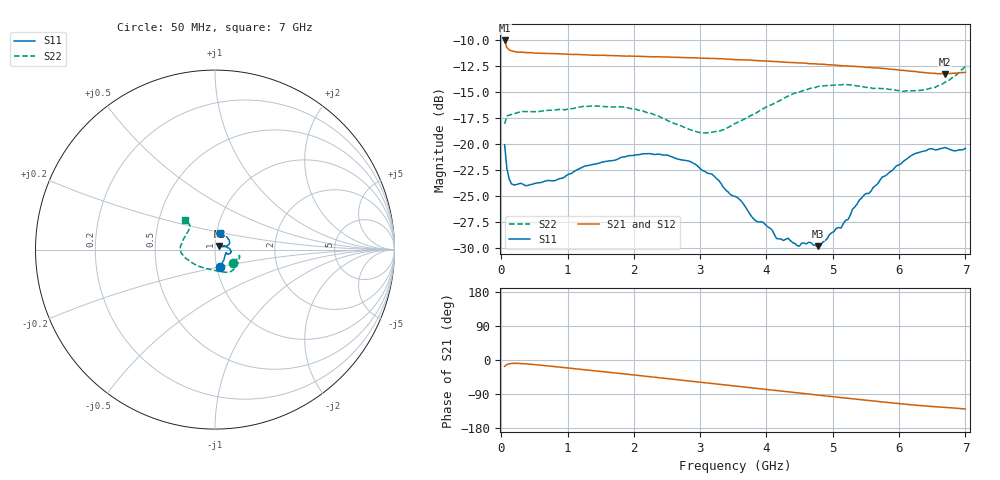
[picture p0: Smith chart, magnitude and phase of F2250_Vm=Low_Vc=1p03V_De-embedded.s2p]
! Integrated Device Technology
! Corporate Headquarters
! 6024 Silver Creek Valley Road
! San Jose, CA 95138  USA
! Phone:  1-408-284-8200
! Toll Free:  1-800-223-1366
! Webpage:  http://www.idt.com/
! Timing and RF Division
! 515 Groton Road, Suite 102
! Westford, MA 01886-6024
! Device:  F2250
! Description: Voltage Variable RF Attenuator
! Frequency:  50.0 -  6000.00 MHz
! Package:  3x3 mm Thin QFN Plastic Package: 16 pin
! Ports:  2 RF, 3 DC
!  Pin  1  = GND
!  Pin  2  = NC
!  Pin  3  = RF1  = Port 1
!  Pin  4  = NC
!  Pin  5  = GND
!  Pin  6  = GND
!  Pin  7  = GND
!  Pin  8  = GND
!  Pin  9  = NC
!  Pin 10  = RF2  = Port 2
!  Pin 11  = NC
!  Pin 12  = GND
!  Pin 13  = GND
!  Pin 14  = VCNTRL
!  Pin 15  = VDD
!  Pin 16  = VMODE
! Vcntrl:  1.030 Volts
! Vmode:  +0.000 Volts
! Vdd:  +3.30  Volts
! Current:  1.188 mA
! Data:  The device was measured on a the F2250 evaluation board which has
!  individual transmission lines to the RF pins.  Data was collected
!  using a calibrated network analyzer.  The evaluation board was
!  de-embedded using a TRL calibration technique.
!  The reference plane is the edge of the package pin.
! Misc:  SN 10
!  Action Tracker AT0258
! Date Measured:  2014-11-26
! Date:  2015-10-15  MJV
! Note:
!  Integrated Device Technology supplies this data as a sample of measured
!  data at the package pin for this product.  Your particular data for this
!  product may vary.
!  Data was taken at 25 degrees C.
!  Integrated Device Technology reserves the right to change this data at anytime.
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# GHz S dB R 50
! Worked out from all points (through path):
!   201 points, 50 MHz to 7 GHz, reference 50 ohm
!   highest |S21| = -10.00 dB at 50 MHz (marker M1); lowest = -13.2 dB at 6.687 GHz (marker M2)
!   group delay of S21, straight-line fit = 51.3 ps
!   lowest |S11| = -29.8 dB at 4.776 GHz (marker M3), VSWR 1.07, Z = 52.5 + j2.14 ohm
!   |S11| at or under -10 dB: start of sweep to end of sweep
!   |S22| runs from -18.9 to -12.5 dB; largest |S21 - S12| = 0.00076
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0.05  -20.05 -73.6  -10.00 -16.6  -10.01 -16.6  -18.05 -35.6
0.08475  -22.37 -49.6  -10.69 -11.9  -10.71 -11.9  -17.29 -19.9
0.1195  -23.37 -38.6  -10.92 -10.0  -10.93 -10.0  -17.19 -15.2
0.189  -23.94 -26.4  -11.06 -8.8  -11.07 -8.8  -17.07 -13.5
0.8145  -23.51 -16.6  -11.28 -17.6  -11.27 -17.6  -16.70 -29.3
1.2315  -22.20 -18.7  -11.37 -25.2  -11.37 -25.2  -16.37 -40.9
1.857  -21.23 -13.8  -11.51 -36.8  -11.51 -36.8  -16.43 -54.4
2.37825  -20.96 -6.7  -11.57 -46.6  -11.59 -46.6  -17.31 -67.5
2.86475  -21.72 3.3  -11.67 -55.9  -11.67 -55.9  -18.63 -88.9
3.0385  -22.55 6.9  -11.71 -59.3  -11.71 -59.3  -18.92 -99.3
3.525  -25.03 18.9  -11.85 -68.7  -11.85 -68.7  -18.02 -129.8
3.803  -27.19 29.1  -11.93 -74.0  -11.93 -74.0  -17.12 -143.7
4.081  -28.25 39.2  -12.03 -79.4  -12.03 -79.4  -16.19 -155.9
4.1505  -29.09 40.4  -12.04 -80.7  -12.03 -80.7  -15.95 -158.4
4.7065  -29.71 41.9  -12.26 -91.3  -12.25 -91.3  -14.59 -173.2
4.776  -29.84 39.2  -12.29 -92.6  -12.28 -92.6  -14.44 -174.6
5.1235  -28.10 27.2  -12.43 -99.2  -12.42 -99.2  -14.29 177.6
5.4015  -25.39 19.2  -12.53 -104.3  -12.53 -104.4  -14.41 171.2
5.85325  -22.71 17.8  -12.76 -112.5  -12.77 -112.5  -14.72 159.8
6.2355  -20.92 24.9  -12.99 -119.0  -12.99 -119.0  -14.86 147.2
6.68725  -20.32 45.2  -13.22 -125.0  -13.22 -125.0  -14.04 135.5
7  -20.41 72.0  -13.08 -129.3  -13.06 -129.4  -12.50 135.5
